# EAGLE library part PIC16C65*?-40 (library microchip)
MICROCONTROLLER
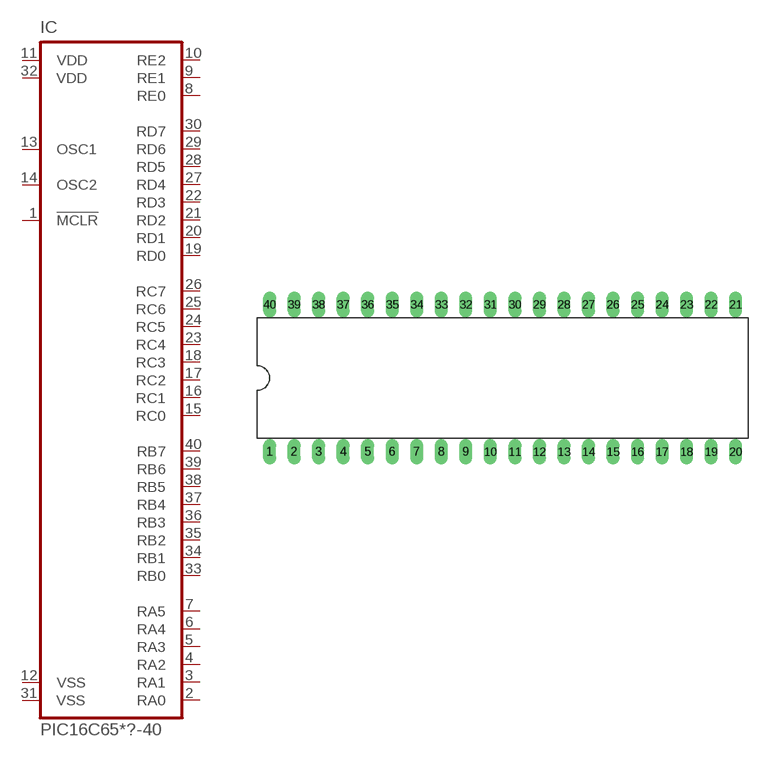
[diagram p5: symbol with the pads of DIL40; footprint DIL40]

Designator prefix IC

## PIC16C65P-40 (MF: MICROCHIP; MPN: PIC16C65B-20/P; OC_FARNELL: 9759670; OC_NEWARK: 12C1910), PIC16C65AP-40 (MPN: PIC16C65A-04/P; OC_FARNELL: 9759670; OC_NEWARK: 97K7249), PIC16C65BP-40 (MF: MICROCHIP; MPN: PIC16C65B-04/P; OC_FARNELL: 9759719; OC_NEWARK: 23C4232)  [DIL40]
1  !MCLR  in
2  RA0
3  RA1
4  RA2
5  RA3
6  RA4
7  RA5
8  RE0
9  RE1
10  RE2
11  VDD  pwr
12  VSS  pwr
13  OSC1  in
14  OSC2  out
15  RC0  out
16  RC1  out
17  RC2  out
18  RC3  out
19  RD0
20  RD1
21  RD2
22  RD3
23  RC4  out
24  RC5  out
25  RC6  out
26  RC7  out
27  RD4
28  RD5
29  RD6
30  RD7
31  VSS  pwr
32  VDD  pwr
33  RB0
34  RB1
35  RB2
36  RB3
37  RB4
38  RB5
39  RB6
40  RB7

## PIC16C65JW-40 (MPN: PIC16C65A-04/P; OC_FARNELL: unknown; OC_NEWARK: 97K7249), PIC16C65AJW-40 (MPN: PIC16C65A-04/P; OC_FARNELL: 9759670; OC_NEWARK: 97K7249), PIC16C65BJW-40 (MF: MICROCHIP; MPN: PIC16C65B/JW; OC_FARNELL: 9759719; OC_NEWARK: 96K3817)  [DIL40]
Pads as for DIL40

## Footprint DIL40 (pad centres in mm)
Dual In Line package type P
drill 0.813 long: 1 -24.13,-7.62; 2 -21.59,-7.62; 3 -19.05,-7.62; 4 -16.51,-7.62; 5 -13.97,-7.62; 6 -11.43,-7.62; 7 -8.89,-7.62; 8 -6.35,-7.62; 9 -3.81,-7.62; 10 -1.27,-7.62; 11 1.27,-7.62; 12 3.81,-7.62; 13 6.35,-7.62; 14 8.89,-7.62; 15 11.43,-7.62; 16 13.97,-7.62; 17 16.51,-7.62; 18 19.05,-7.62; 19 21.59,-7.62; 20 24.13,-7.62; 21 24.13,7.62; 22 21.59,7.62; 23 19.05,7.62; 24 16.51,7.62; 25 13.97,7.62; 26 11.43,7.62; 27 8.89,7.62; 28 6.35,7.62; 29 3.81,7.62; 30 1.27,7.62; 31 -1.27,7.62; 32 -3.81,7.62; 33 -6.35,7.62; 34 -8.89,7.62; 35 -11.43,7.62; 36 -13.97,7.62; 37 -16.51,7.62; 38 -19.05,7.62; 39 -21.59,7.62; 40 -24.13,7.62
